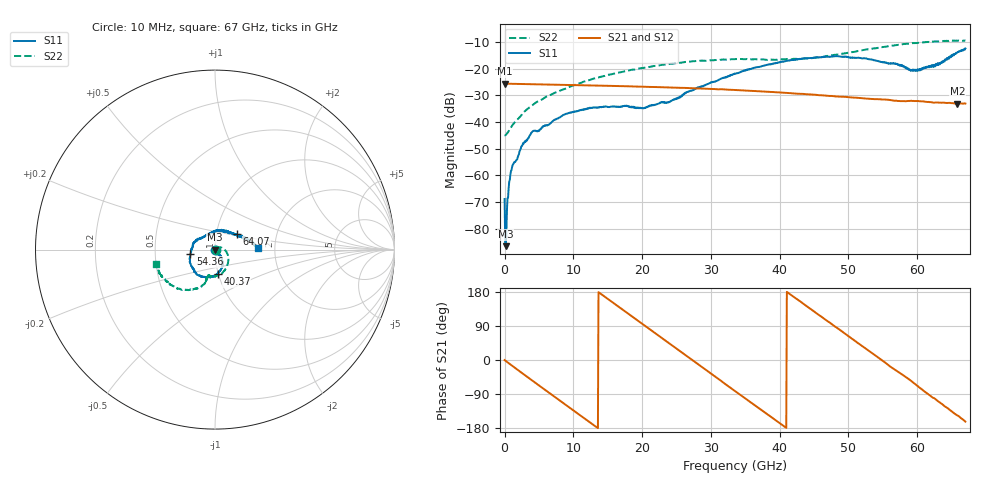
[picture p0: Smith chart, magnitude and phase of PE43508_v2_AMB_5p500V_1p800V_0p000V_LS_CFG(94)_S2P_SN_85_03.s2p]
!Keysight Technologies,N5227A,US51270237,A.10.43.00
!Date: Wednesday, August 22, 2018 17:16:28
!Correction: S11(Full 2 Port(1,3))
!S31(Full 2 Port(1,3))
!S13(Full 2 Port(1,3))
!S33(Full 2 Port(1,3))
!S2P File: Measurements: S11, S31, S13, S33:
# Hz S  dB  R 50
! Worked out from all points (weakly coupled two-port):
!   801 points, 10 MHz to 67 GHz, reference 50 ohm
!   highest |S21| = -25.57 dB at 10 MHz (marker M1); lowest = -33.1 dB at 65.83 GHz (marker M2)
!   lowest |S11| = -86.5 dB at 177.5 MHz (marker M3), VSWR 1.00, Z = 50 + j0.00422 ohm
!   |S11| at or under -10 dB: start of sweep to end of sweep
!   |S22| runs from -45.0 to -9.4 dB; largest |S21 - S12| = 0.00026
!   S11 on the Smith chart (normalised r, x): 10 MHz: 1.00, -0.00; 40.37 GHz: 0.99, -0.27; 54.36 GHz: 0.76, -0.04; 64.07 GHz: 1.26, +0.22; 67 GHz: 1.63, +0.03
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1e7  -68.84 -67.3  -25.57 -0.2  -25.57 -0.2  -44.88 -1.5
1.77475e8  -86.49 63.0  -25.59 -2.6  -25.60 -2.6  -44.79 8.4
4.286875e8  -68.50 -8.4  -25.61 -6.0  -25.62 -6.0  -44.02 17.4
7.636375e8  -61.66 -22.6  -25.63 -10.6  -25.63 -10.6  -42.75 25.0
1.098588e9  -56.82 -21.5  -25.65 -15.1  -25.65 -15.1  -41.35 30.0
2.773338e9  -48.07 -42.2  -25.74 -37.6  -25.75 -37.6  -36.41 36.5
4.196875e9  -43.29 -47.6  -25.82 -56.4  -25.82 -56.4  -33.37 32.4
8.7187e9  -37.11 -76.8  -26.05 -116.1  -26.05 -116.1  -27.63 11.9
1.123082e10  -35.33 -83.1  -26.18 -149.1  -26.19 -149.1  -25.13 -2.6
1.759488e10  -33.97 -89.1  -26.56 127.3  -26.56 127.3  -20.92 -34.4
2.019074e10  -34.75 -80.5  -26.75 93.1  -26.75 93.1  -19.68 -45.6
2.236791e10  -33.02 -68.3  -26.90 64.5  -26.90 64.5  -18.80 -55.2
3.3505e10  -21.89 -59.8  -27.97 -82.0  -27.97 -82.0  -16.41 -93.9
4.037148e10  -17.35 -83.9  -28.96 -171.6  -28.94 -171.6  -16.46 -104.8
4.472582e10  -15.95 -106.1  -29.66 131.7  -29.65 131.7  -16.04 -105.2
4.841028e10  -15.28 -125.8  -30.41 83.8  -30.41 83.8  -14.72 -105.9
5.435564e10  -17.13 -170.0  -31.43 6.4  -31.41 6.2  -12.14 -117.9
5.586291e10  -18.15 172.7  -31.65 -14.4  -31.62 -14.8  -11.49 -122.2
5.979858e10  -20.35 114.5  -32.09 -64.8  -32.09 -65.1  -10.39 -135.8
6.406919e10  -16.48 35.5  -32.82 -123.3  -32.86 -123.5  -9.64 -153.6
6.582768e10  -13.89 14.8  -33.13 -146.3  -33.20 -146.5  -9.50 -160.1
6.7e10  -12.40 1.9  -33.04 -162.6  -33.10 -162.6  -9.44 -166.4
